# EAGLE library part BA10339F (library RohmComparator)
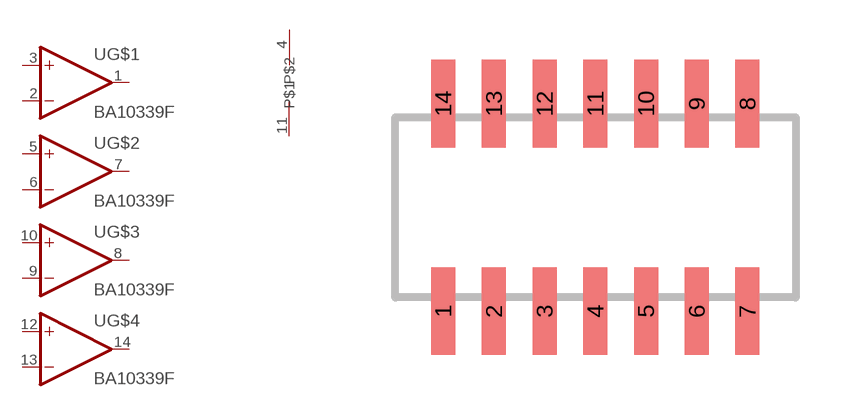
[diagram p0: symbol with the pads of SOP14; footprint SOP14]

Designator prefix -; gates G$5=SUPPLY G$1=OPAMP G$2=OPAMP G$3=OPAMP G$4=OPAMP

## BA10339F  [SOP14]
1  G$1:OUT  out
2  G$1:-IN  in
3  G$1:+IN  in
4  G$5:P$1
5  G$2:+IN  in
6  G$2:-IN  in
7  G$2:OUT  out
8  G$3:OUT  out
9  G$3:-IN  in
10  G$3:+IN  in
11  G$5:P$2
12  G$4:+IN  in
13  G$4:-IN  in
14  G$4:OUT  out

## Footprint SOP14 (pad centres in mm)
smd 0.6 x 2.2: 1 -3.81,-2.6; 2 -2.54,-2.6; 3 -1.27,-2.6; 4 0,-2.6; 5 1.27,-2.6; 6 2.54,-2.6; 7 3.81,-2.6; 8 3.81,2.6; 9 2.54,2.6; 10 1.27,2.6; 11 0,2.6; 12 -1.27,2.6; 13 -2.54,2.6; 14 -3.81,2.6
